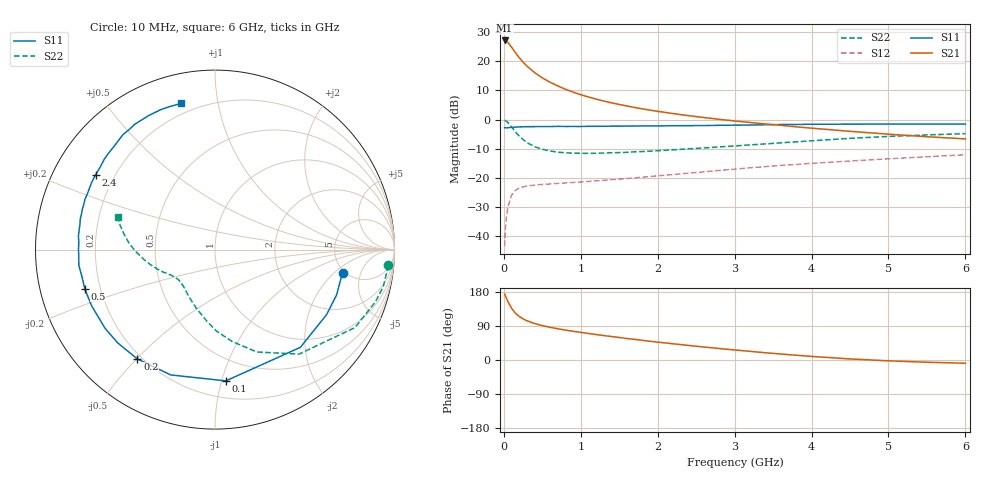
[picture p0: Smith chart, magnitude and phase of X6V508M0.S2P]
! SIEMENS Small Signal Semiconductors
! BFP193W
! Si NPN RF Bipolar Junction Transistor in SOT343
! VCE = 0.5 V  IC = 8 mA
! Common Emitter S-Parameters:  April 1994
# GHz  S  MA  R  50
!  f  S11  S21  S12  S22
! GHz  MAG  ANG  MAG  ANG  MAG  ANG  MAG  ANG
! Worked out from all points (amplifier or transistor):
!   40 points, 10 MHz to 6 GHz, reference 50 ohm
!   highest |S21| = 27.1 dB at 10 MHz (marker M1)
!   |S21| within 3 dB of that: start of sweep to 119.5 MHz
!   unconditionally stable (mu >= 1): 1.238 GHz to end of sweep
!   at 200 MHz: K = 0.21, MSG = 22.3 dB, |S12| = -23.5 dB
!   at 1.5 GHz: K = 1.11, MAG = 10.8 dB, |S12| = -20.4 dB
!   at 6 GHz: K = 1.11, MAG = 0.7 dB, |S12| = -12.1 dB
!   S11 on the Smith chart (normalised r, x): 10 MHz: 4.78, -2.56; 100 MHz: 0.33, -1.03; 200 MHz: 0.18, -0.50; 500 MHz: 0.14, -0.14; 2.4 GHz: 0.13, +0.28; 6 GHz: 0.14, +0.78
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0.01  0.7221 -10.2  22.53 174.1  0.0068 84.6  0.9702 -5.2
0.02  0.7229 -20.4  22.45 169.8  0.0134 80.8  0.9601 -12.3
0.03  0.7196 -30.2  22.12 164.8  0.0196 75.4  0.9403 -18.0
0.05  0.723 -48.9  20.96 155.3  0.0308 67.6  0.8929 -29.1
0.1  0.7339 -85.3  17.34 136.7  0.0503 50.6  0.7472 -51.2
0.15  0.7407 -109.5  14 123.6  0.0613 40.4  0.6161 -67.8
0.2  0.7471 -125.4  11.44 114.8  0.0669 34.0  0.5196 -79.6
0.25  0.751 -136.1  9.621 108.5  0.0704 29.6  0.4544 -88.9
0.3  0.7533 -144.3  8.204 103.6  0.0728 27.3  0.4031 -96.2
0.4  0.7556 -155.6  6.345 96.2  0.0754 24.2  0.3431 -107.6
0.5  0.7579 -163.3  5.161 90.7  0.0776 23.2  0.31 -115.8
0.6  0.7566 -168.8  4.337 86.3  0.0789 22.8  0.2894 -122.5
0.8  0.7598 -177.1  3.295 79.0  0.0821 24.0  0.2693 -131.2
1.1  0.7648 174.4  2.431 70.0  0.0874 26.4  0.2632 -139.3
1.3  0.7657 169.2  2.068 64.4  0.0912 28.3  0.2667 -142.8
1.6  0.7728 163.0  1.703 56.7  0.0979 31.0  0.2744 -147.0
2.2  0.7824 151.5  1.264 42.8  0.1145 34.9  0.3029 -154.5
2.4  0.785 147.9  1.163 38.4  0.1206 35.5  0.3149 -156.5
3.2  0.804 134.5  0.89 22.9  0.149 36.3  0.3677 -166.6
4.5  0.8329 116.6  0.628 2.8  0.1949 32.2  0.4762 176.4
5.5  0.8358 107.5  0.507 -5.9  0.2308 27.8  0.5446 165.8
6  0.836 103.1  0.466 -8.5  0.2493 25.5  0.5723 161.5
